FUNCTION_BLOCK FB_Cylinder IMPLEMENTS ICylinder
(* FB_Cylinder	- number of control signals
						one direction is controllable
				- type of feedback signal
						feedback in base and work position			*)
VAR_INPUT
	bAtBasePos		AT %I*: BOOL;
	bAtWorkPos		AT %I*: BOOL;
END_VAR
VAR_OUTPUT
	bMoveToWork		: BOOL;
END_VAR

// =========================================================
;
// =========================================================

METHOD M_MoveToBase : BOOL
VAR_INPUT
END_VAR
// =========================================================
	// Move to base position
	
M_MoveToBase := M_StateMachine(	bBasePosReq := TRUE,
								bWorkPosReq	:= FALSE );
								
// =========================================================
END_METHOD

PROPERTY PUBLIC P_AtWorkPos : BOOL
SET
END_SET
GET
P_AtWorkPos := bAtWorkPos;
END_GET
END_PROPERTY

PROPERTY PUBLIC P_ToWork : BOOL
GET
P_ToWork := bMoveToWork;
END_GET
SET
END_SET
END_PROPERTY

METHOD M_MoveToWork : BOOL
VAR_INPUT
END_VAR
// =========================================================
	// Move to work position
	
M_MoveToWork := M_StateMachine(	bBasePosReq := FALSE,
								bWorkPosReq	:= TRUE );
								
// =========================================================
END_METHOD

PROPERTY PUBLIC P_AtBasePos : BOOL
SET
END_SET
GET
P_AtBasePos := bAtBasePos;
END_GET
END_PROPERTY

METHOD M_StateMachine : BOOL
VAR_INPUT
	bBasePosReq		: BOOL;
	bWorkPosReq		: BOOL;
END_VAR
// =========================================================
		// Base or work position requested
		
IF bWorkPosReq THEN
	bMoveToWork := TRUE;
END_IF

IF bBasePosReq OR NOT bWorkPosReq THEN
	bMoveToWork := FALSE;
END_IF

// =========================================================
	// Return
	
M_StateMachine := FALSE;

// =========================================================
END_METHOD

METHOD PUBLIC M_Reset
VAR_INPUT
END_VAR
// =========================================================
	// Reset
	
bMoveToWork := FALSE;

// =========================================================
END_METHOD

END_FUNCTION_BLOCK
